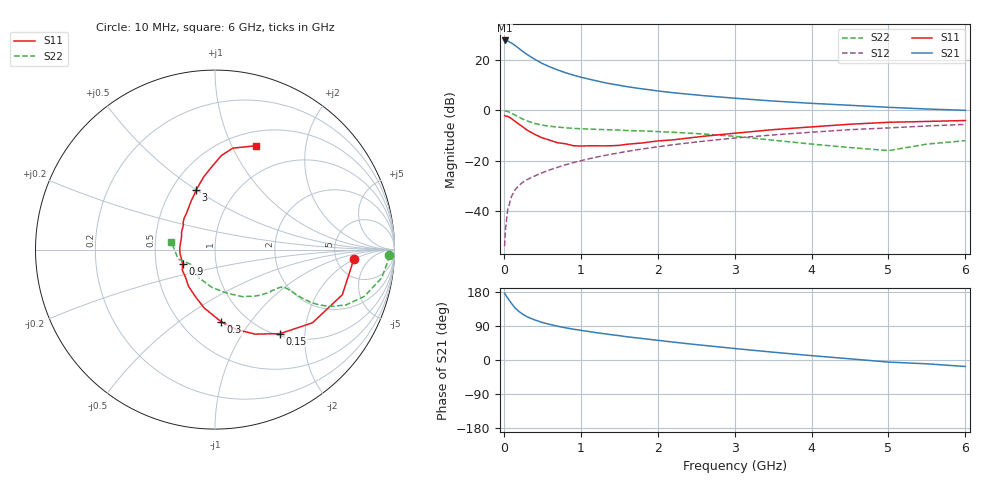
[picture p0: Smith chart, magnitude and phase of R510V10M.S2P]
! SIEMENS Small Signal Semiconductors
! BFR183
! Si NPN RF Bipolar Junction Transistor in SOT23
! VCE = 10 V  IC = 10 mA
! Common Emitter S-Parameters:  May  1996
# GHz  S  MA  R  50
!  f  S11  S21  S12  S22
! GHz  MAG  ANG  MAG  ANG  MAG  ANG  MAG  ANG
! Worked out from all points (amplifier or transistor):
!   36 points, 10 MHz to 6 GHz, reference 50 ohm
!   highest |S21| = 27.6 dB at 10 MHz (marker M1)
!   |S21| within 3 dB of that: start of sweep to 188.8 MHz
!   unconditionally stable (mu >= 1): 846.5 MHz to 2.646 GHz
!   at 250 MHz: K = 0.60, MSG = 25.9 dB, |S12| = -28.5 dB
!   at 1.4 GHz: K = 1.05, MAG = 12.6 dB, |S12| = -17.5 dB
!   at 6 GHz: K = 0.89, MSG = 2.8 dB, |S12| = -5.6 dB
!   S11 on the Smith chart (normalised r, x): 10 MHz: 7.37, -1.94; 150 MHz: 1.04, -1.50; 300 MHz: 0.77, -0.74; 900 MHz: 0.69, -0.11; 3 GHz: 0.66, +0.50; 6 GHz: 0.66, +1.24
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0.01  0.775 -3.9  24.12 176.0  0.002 78.8  0.9705 -1.9
0.02  0.7641 -8.0  24.1 172.6  0.0041 81.1  0.9651 -3.9
0.05  0.7526 -19.5  23.61 163.3  0.0105 79.1  0.9424 -9.6
0.1  0.6792 -36.9  21.37 149.2  0.0195 72.3  0.8719 -17.4
0.15  0.5924 -52.2  18.96 136.4  0.0267 67.6  0.7923 -22.9
0.2  0.5218 -64.5  16.57 127.5  0.0325 64.7  0.7192 -26.1
0.25  0.4611 -75.1  14.45 120.2  0.0374 63.1  0.6604 -27.9
0.3  0.4037 -85.0  12.77 114.2  0.0417 63.2  0.6131 -28.8
0.4  0.331 -100.5  10.26 105.9  0.0492 63.0  0.5452 -29.1
0.5  0.282 -113.2  8.414 99.1  0.0575 63.4  0.5037 -28.8
0.6  0.2525 -125.7  7.193 93.8  0.0655 63.9  0.4794 -28.6
0.7  0.2252 -136.9  6.28 89.1  0.0736 64.8  0.4611 -28.5
0.9  0.1972 -156.5  4.958 81.5  0.091 64.9  0.4353 -28.6
1.1  0.1963 -174.1  4.143 75.3  0.1078 64.7  0.4216 -30.0
1.3  0.1955 170.2  3.534 69.4  0.1253 64.0  0.4107 -31.5
1.6  0.2101 152.3  2.927 61.3  0.1517 62.2  0.3947 -34.9
2.2  0.2575 128.0  2.215 47.3  0.2058 57.6  0.364 -43.6
3  0.3476 107.8  1.725 30.3  0.2795 49.3  0.3032 -59.8
3.5  0.4101 98.8  1.515 20.6  0.322 43.2  0.2535 -74.0
4.5  0.5254 86.1  1.247 3.1  0.4098 31.5  0.181 -119.6
5.5  0.5967 73.6  1.053 -10.1  0.4851 20.2  0.2118 -165.7
6  0.6223 68.5  0.99 -17.1  0.5218 12.7  0.2479 169.6
